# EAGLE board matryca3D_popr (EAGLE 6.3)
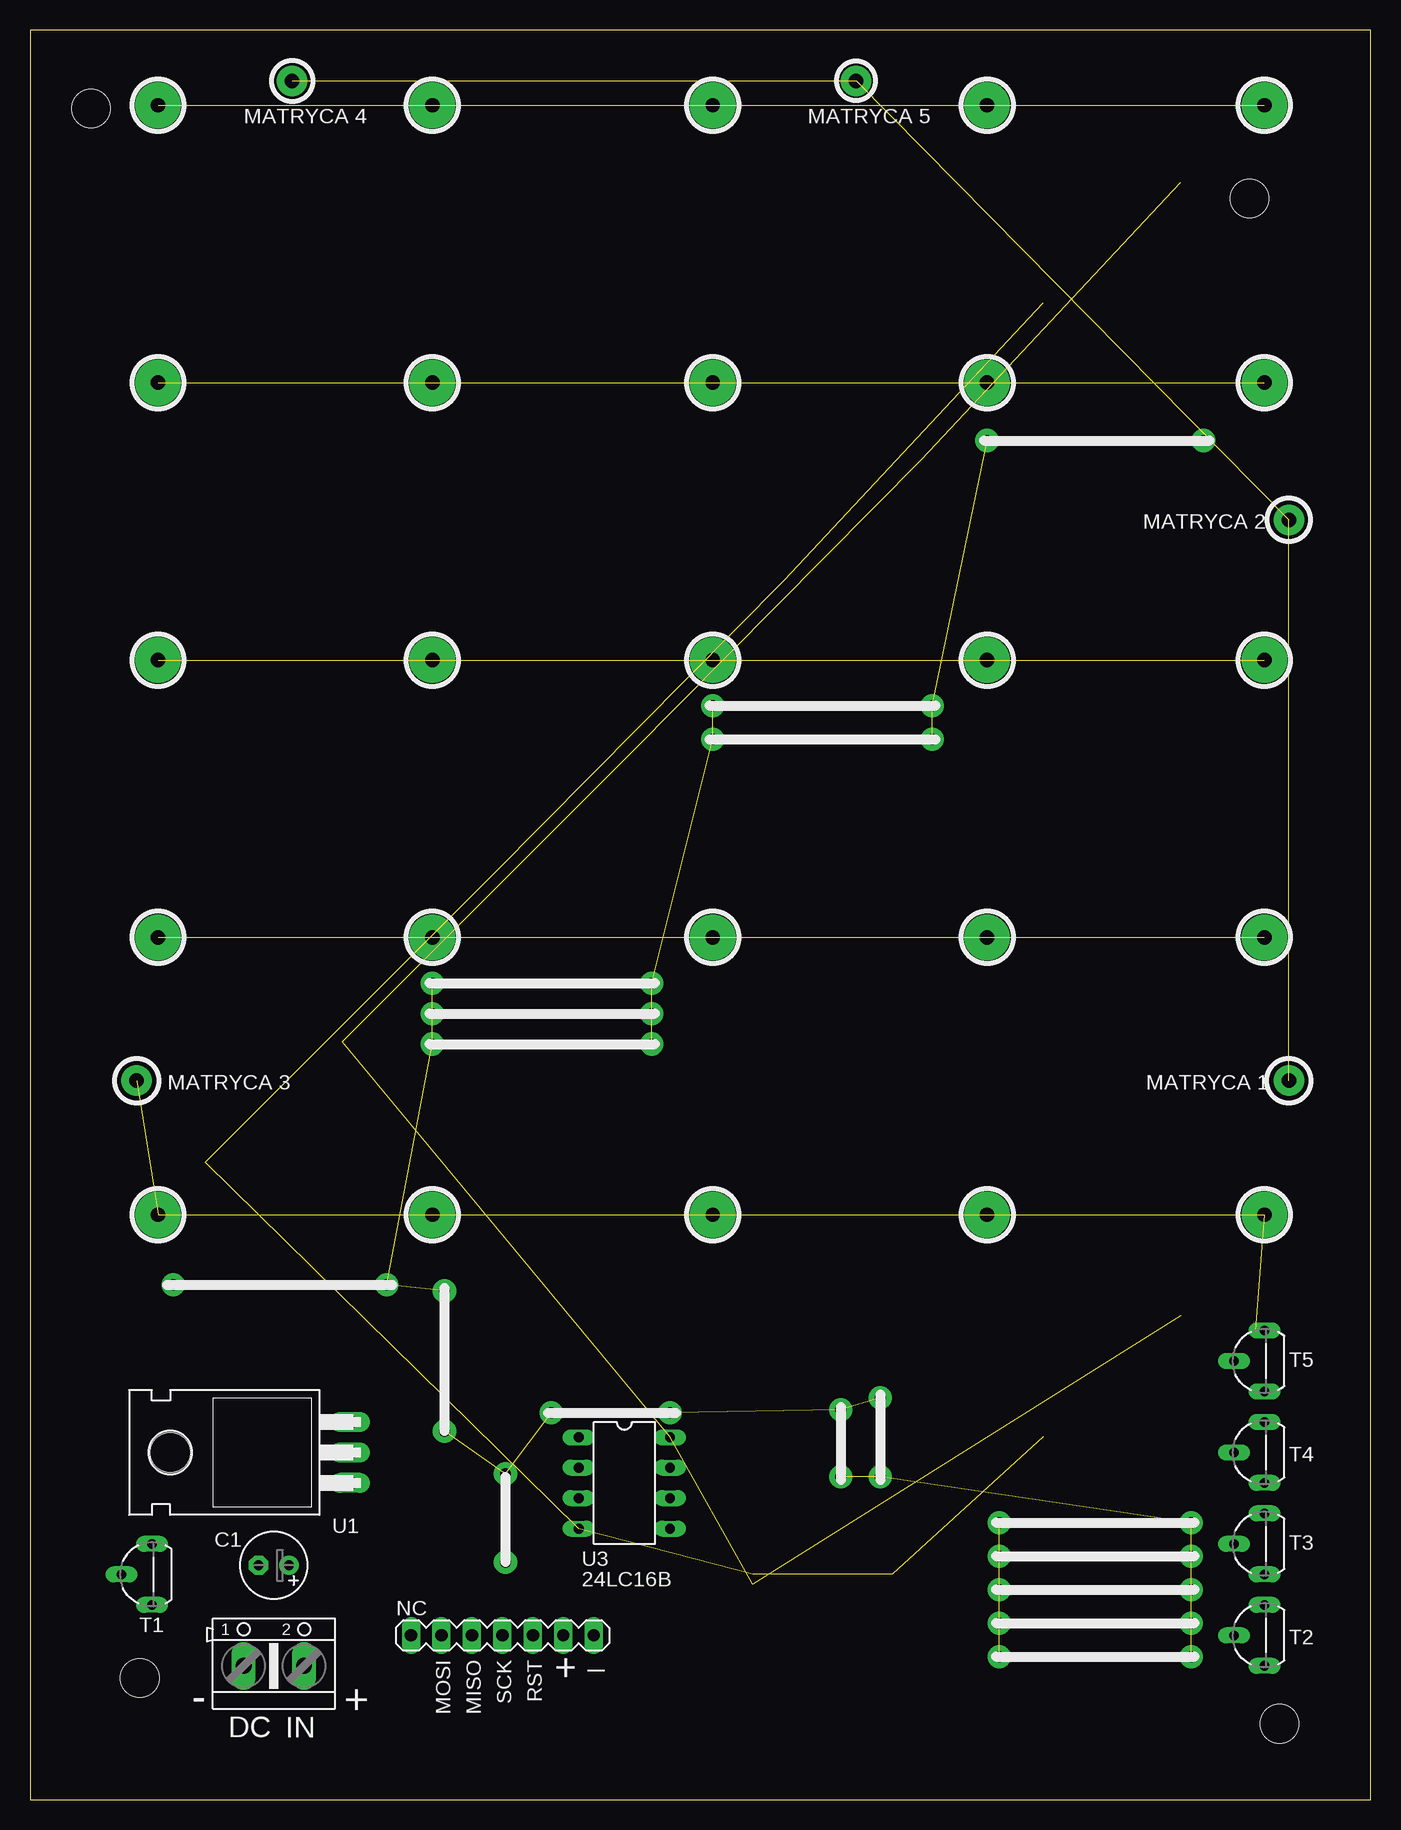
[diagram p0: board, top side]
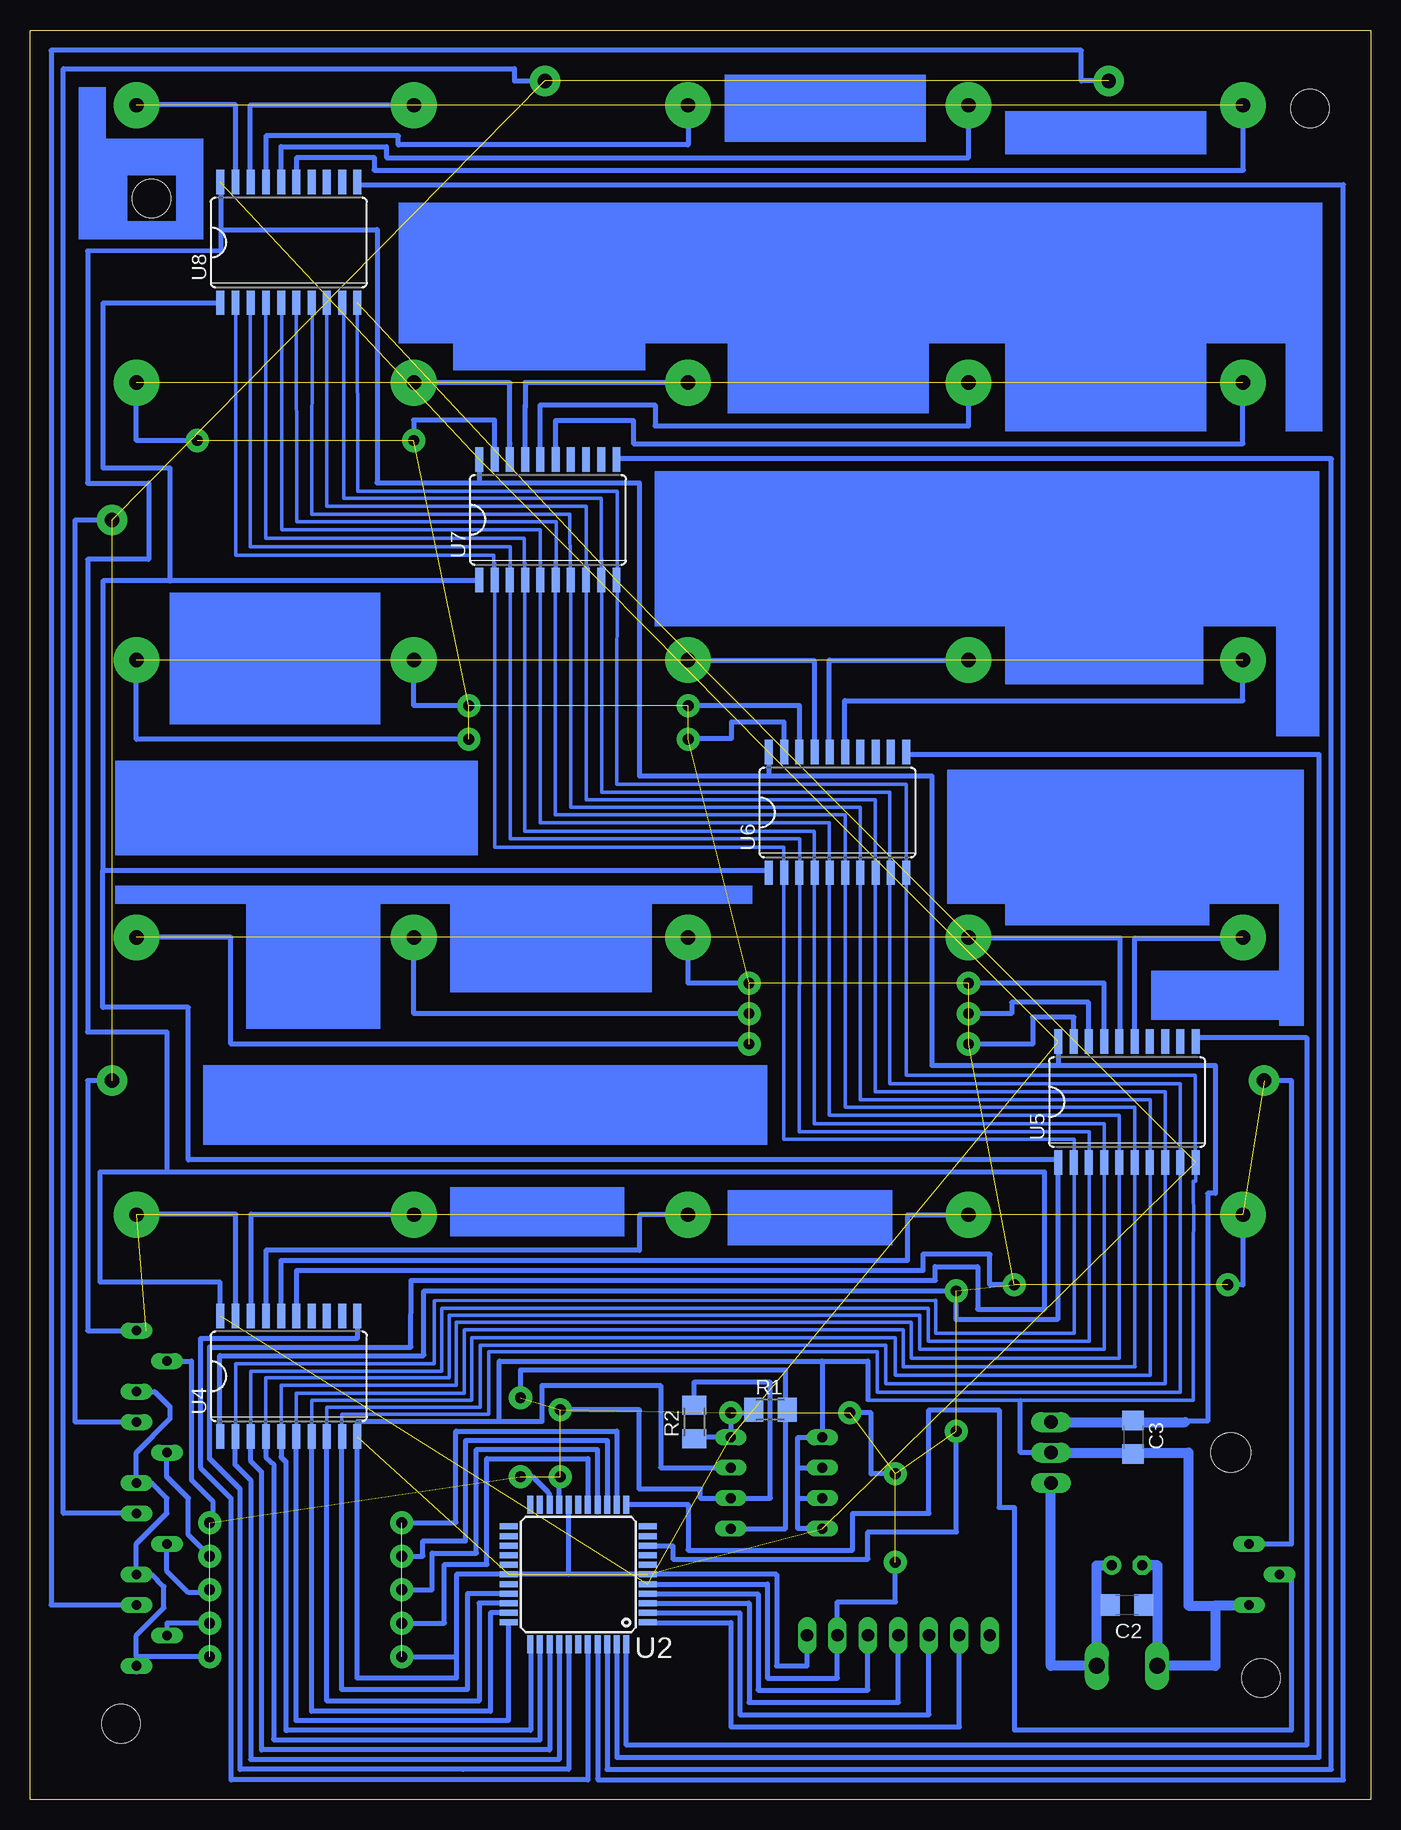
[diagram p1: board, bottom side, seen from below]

Size 111.74 x 147.5 mm. Coordinates in mm from the lower left corner, seen from the top.
Outline: 0,0 111.74,0 111.74,147.5 0,147.5 0,0
Copper layers (1*16): Top 0.035mm / dielectric 1.5mm / Bottom 0.035mm
Design rules "default": minimum track width 10mil, minimum drill 24mil, track to track 8mil, track to pad 8mil, pad to pad 8mil, via to via 8mil, smd to smd 8mil, copper to edge 40mil, drill to drill 8mil, minimum pad ring 10mil, minimum via ring 8mil, stop-mask expansion 4mil, vias tented up to drill 0mil, thermal gap 10mil
Holes 3.2 mm at 9.14,10.16 104.14,6.35 101.63,133.45 5.08,140.97

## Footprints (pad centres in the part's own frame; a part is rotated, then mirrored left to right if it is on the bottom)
E2,5-6 = drill 0.813 pad 1.6: + -1.27,0 | drill 0.813 pad 1.6 octagon: - 1.27,0
C1206 = smd 1.6 x 1.8: 1 -1.4,0; 2 1.4,0
AK500/2 = drill 1.321 long: 1 -2.515,0; 2 2.515,0
MA07-1 = drill 1.016 long: 1 -7.62,0; 2 -5.08,0; 3 -2.54,0; 4 0,0; 5 2.54,0; 6 5.08,0; 7 7.62,0
M1206 = smd 1.6 x 2: 1 -1.4,0; 2 1.4,0
TO92L = drill 0.813 long: 1 0,-2.54; 2 2.54,0; 3 0,2.54
TO220H = drill 1.118 long: 1 -2.54,-10.16; 2 0,-10.16; 3 2.54,-10.16 | hole 3.302: 0,4.826
TQFP44 = smd 1.5 x 0.5: 1 -5.8,4; 2 -5.8,3.2; 3 -5.8,2.4; 4 -5.8,1.6; 5 -5.8,0.8; 6 -5.8,0; 7 -5.8,-0.8; 8 -5.8,-1.6; 9 -5.8,-2.4; 10 -5.8,-3.2; 11 -5.8,-4; 23 5.8,-4; 24 5.8,-3.2; 25 5.8,-2.4; 26 5.8,-1.6; 27 5.8,-0.8; 28 5.8,0; 29 5.8,0.8; 30 5.8,1.6; 31 5.8,2.4; 32 5.8,3.2; 33 5.8,4 | smd 0.5 x 1.5: 12 -4,-5.8; 13 -3.2,-5.8; 14 -2.4,-5.8; 15 -1.6,-5.8; 16 -0.8,-5.8; 17 0,-5.8; 18 0.8,-5.8; 19 1.6,-5.8; 20 2.4,-5.8; 21 3.2,-5.8; 22 4,-5.8; 34 4,5.8; 35 3.2,5.8; 36 2.4,5.8; 37 1.6,5.8; 38 0.8,5.8; 39 0,5.8; 40 -0.8,5.8; 41 -1.6,5.8; 42 -2.4,5.8; 43 -3.2,5.8; 44 -4,5.8
DIL8 = drill 0.813 long: 1 -3.81,-3.81; 2 -1.27,-3.81; 3 1.27,-3.81; 4 3.81,-3.81; 5 3.81,3.81; 6 1.27,3.81; 7 -1.27,3.81; 8 -3.81,3.81
SO20W = smd 0.66 x 2.032: 1 -5.715,-5.029; 2 -4.445,-5.029; 3 -3.175,-5.029; 4 -1.905,-5.029; 5 -0.635,-5.029; 6 0.635,-5.029; 7 1.905,-5.029; 8 3.175,-5.029; 9 4.445,-5.029; 10 5.715,-5.029; 11 5.715,5.029; 12 4.445,5.029; 13 3.175,5.029; 14 1.905,5.029; 15 0.635,5.029; 16 -0.635,5.029; 17 -1.905,5.029; 18 -3.175,5.029; 19 -4.445,5.029; 20 -5.715,5.029

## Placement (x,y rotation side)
C1  [E2,5-6]  20.32,19.56 180 top
C2  [C1206]  20.32,16.26 0 bottom
C3  [C1206]  19.81,30.23 270 bottom
DC  [AK500/2]  20.32,11.18 0 top
NC  [MA07-1]  39.37,13.72 0 top
R1  [M1206]  50.04,32.51 0 bottom
R2  [M1206]  56.39,31.5 90 bottom
T1  [TO92L]  10.16,18.8 180 top
T2  [TO92L]  102.87,13.72 180 top
T3  [TO92L]  102.87,21.34 180 top
T4  [TO92L]  102.87,28.96 180 top
T5  [TO92L]  102.87,36.58 180 top
U1  7805T  [TO220H]  16.51,28.96 90 top
U2  MEGA32-A  [TQFP44]  66.04,18.8 180 bottom
U3  24LC16BP  [DIL8]  49.53,26.42 270 top
U4  74HCT574D  [SO20W]  90.17,35.31 0 bottom
U5  74HCT574D  [SO20W]  20.32,58.17 0 bottom
U6  74HCT574D  [SO20W]  44.45,82.3 0 bottom
U7  74HCT574D  [SO20W]  68.58,106.68 0 bottom
U8  74HCT574D  [SO20W]  90.17,129.79 0 bottom

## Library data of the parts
C1-C3 R1 R2 = rcl
DC = con-ptr500; OC_FARNELL: unknown; OC_NEWARK: unknown
NC = con-lstb; OC_FARNELL: unknown; OC_NEWARK: unknown
T1-T5 = transistor
U1 = linear
U2 = atmel; MPN: ATMEGA32-16AU; OC_FARNELL: 9171274; OC_NEWARK: 69K6677
U3 = microchip; MF: MICROCHIP; MPN: 24LC16B/P; OC_FARNELL: 1200026; OC_NEWARK: 69K7671
U4-U8 = 74xx-eu

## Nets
AVCC: U2.27
GND: U2.6 U2.28 U3.4 U4.10 U5.10 U6.10 U7.10 U8.10
GND1: U2.18
GND2: U2.39
VCC: U2.5 U3.8 U4.20 U5.20 U6.20 U7.20 U8.20
VCC1: U2.17
VCC2: U2.38

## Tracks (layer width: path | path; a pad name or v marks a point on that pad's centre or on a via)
GND  (7 unrouted)
N$1
  Bottom 0.305: 87.02,29.54 87,29.54 87,32.74 74.22,32.74 74.22,37.9 40.41,37.9 40.41,34.67 17.14,34.67 17.14,59 41.3,59 41.3,83.36 65.41,83.36 65.41,102.72
N$2
  Bottom 0.406: 60.48,17.98 50.29,17.98 50.29,10.16 44.45,10.16 44.45,14.73
N$3
  Bottom 0.406: 46.97,12.52 46.99,12.52 46.99,14.73
N$4
  Bottom 0.406: 60.38,17.17 51.05,17.17 51.05,9.14 41.91,9.14 41.91,14.73
N$5
  Bottom 0.406: 60.38,16.41 51.82,16.41 51.82,8.13 39.37,8.13 39.37,14.48
N$6
  Bottom 0.406: 60.43,15.6 52.58,15.6 52.58,7.11 36.83,7.11 36.83,14.73
N$7
  Bottom 0.406: 60.25,14.78 53.34,14.78 53.34,6.1 34.29,6.1 34.29,14.73
N$8  (via drill 0.9 pad 1.93)  (28 unrouted)
  other vias: 39.62,19.81 39.62,27.18 43.43,32.26 34.54,30.73 96.77,23.11 96.77,20.32 96.77,17.53 96.77,14.73 96.77,11.94 79.76,113.28 97.79,113.28 56.9,88.39 56.9,91.19 75.18,91.19 75.18,88.39 33.53,68.07 33.53,65.53 33.53,62.99 51.82,68.07 51.82,65.53 51.82,62.99 67.56,26.92 70.87,26.92 67.56,26.92 67.56,32.51 70.87,33.53 53.34,32.26 34.54,42.42 29.72,42.93 11.94,42.93
N$9
  Bottom 0.305: 89.53,29.84 89.53,33.91 75.56,33.91 75.56,39.17 38.96,39.17 38.96,36.09 19.63,36.09
N$10
  Bottom 0.406: 60.4,21.18 58.17,21.18 58.17,20.07 41.91,20.07 41.91,22.35 34.54,22.35 34.54,31.24
N$11
  Bottom 0.406: 61.98,24.64 56.9,24.64 56.9,20.83 43.18,20.83 43.18,23.88 36.83,23.88 36.83,32.51 30.99,32.51 30.99,24.38 29.72,24.38 29.72,5.84 6.6,5.84 6.6,18.8 8.38,18.8
N$12  (via drill 1.2 pad 3.81)  (4 unrouted)
  other vias: 10.67,141.22 33.53,141.22 56.9,141.22 79.76,141.22 102.87,141.22
N$13
  Bottom 0.813: 10.19,16.2 12.95,16.2 12.95,11.18 17.78,11.18
N$14
  Bottom 0.813: 17.78,11.43 17.78,16.26 | 17.78,16.26 17.78,19.56 | 19.05,16.26 17.78,16.26
N$15
  Bottom 0.813: 17.78,19.56 19.3,19.56
N$16
  Bottom 0.813: 22.81,11.15 22.86,11.15 22.86,19.56 21.34,19.56
N$17
  Bottom 0.813: 21.59,16.26 22.61,16.26
N$18
  Bottom 0.406: 44.48,14.91 44.45,14.91 44.45,16.51 39.62,16.51 39.62,20.32
N$19
  Bottom 0.406: 39.12,27.18 41.66,27.18 41.66,32.26 43.94,32.26
N$20
  Bottom 0.813: 22.35,11.18 26.67,11.18 26.67,26.67
N$21
  Bottom 0.406: 25.4,28.96 29.21,28.96 29.21,33.27
  Bottom 0.813: 27.69,28.96 25.4,28.96 15.21,28.96 15.21,16.2 12.93,16.2
N$22
  Bottom 0.813: 27.69,31.5 15.49,31.5
N$23
  Bottom 0.406: 62.05,13.41 62.05,4.57 5.33,4.57 5.33,63.5 14.48,63.5
N$24
  Bottom 0.406: 62.81,13.49 62.84,13.49 62.84,3.56 4.32,3.56 4.32,87.12 38.71,87.12
N$25
  Bottom 0.406: 63.63,13.46 63.65,13.46 63.65,2.54 3.3,2.54 3.3,111.76 62.99,111.76
N$26
  Bottom 0.406: 64.44,13.39 64.44,1.8 64.41,1.8 64.41,1.68 2.29,1.68 2.29,134.62 84.58,134.62
N$27
  Bottom 0.406: 65.23,13.18 65.25,13.18 65.25,1.68 95,1.68 95,25.15 97.54,27.69 97.54,38.46 84.48,38.46 84.48,41.02
N$28
  Bottom 0.406: 66.85,13.06 66.85,2.54 75.67,2.54
N$29
  Bottom 0.406: 67.64,13.16 67.64,3.35 93.34,3.35
N$30
  Bottom 0.406: 68.45,13.21 68.43,13.21 68.43,4.17 92.43,4.17
N$31
  Bottom 0.406: 69.24,13.16 69.24,4.98 91.39,4.98
N$32
  Bottom 0.406: 70.05,13.16 70.03,13.16 70.03,5.79 90.3,5.79
N$33  (via drill 0.9 pad 1.93)  (4 unrouted)
  other vias: 80.77,23.11 80.77,20.32 80.77,17.53 80.77,14.73 80.77,11.94
N$34
  Bottom 0.406: 96.6,11.94 102.87,11.94 | 102.87,11.94 102.87,10.67 | 102.87,11.94 102.87,13.72 100.58,16 100.58,17.78 101.6,18.8 102.87,18.8 | 102.87,18.8 103.38,18.8 | 102.87,18.8 102.87,21.34 100.33,23.88 100.33,25.15 101.6,26.42 102.87,26.42 | 103.38,26.42 102.87,26.42 | 103.63,34.04 101.35,34.04 100.08,32.77 100.08,31.75 102.87,28.96 102.87,26.42
N$35
  Bottom 0.406: 96.27,17.27 98.55,17.27 100.33,19.05 100.33,21.59
N$36
  Bottom 0.406: 96.27,19.81 98.55,22.1 98.55,25.15 100.33,26.92 100.33,29.21
N$37
  Bottom 0.406: 101.09,36.58 98.3,36.58 98.3,26.67 96.52,24.89 96.52,22.86
N$38
  Bottom 0.406: 102.11,31.5 107.95,31.5 107.95,106.68 103.89,106.68
N$39
  Bottom 0.406: 95.94,30.28 95.91,30.25 95.91,37.03 78.94,37.03
N$40
  Bottom 0.406: 94.67,30.61 94.67,27.96 93.34,26.64 93.34,3.38
N$41
  Bottom 0.406: 93.32,30.76 93.37,30.76 93.37,28.27 92.46,27.36 92.46,4.17
N$42
  Bottom 0.406: 92.05,30.48 92.08,30.48 92.08,28.57 91.44,27.96 91.44,5.08
N$43
  Bottom 0.406: 78.99,37.08 78.92,37.08 78.92,42.42 34.54,42.42
N$44
  Bottom 0.406: 71.88,14.73 71.88,6.6 89.56,6.6 89.56,30.58
N$45
  Bottom 0.406: 96.27,14.73 100.33,14.73 100.33,13.46
N$46
  Bottom 0.406: 71.73,15.6 73.38,15.6 73.38,7.39 88.29,7.39 88.29,30.76 88.27,30.76
N$47
  Bottom 0.406: 71.78,16.41 74.32,16.41 74.32,8.23 87,8.23 87,30.71
N$48
  Bottom 0.305: 92.08,30.58 92.08,35.18 76.81,35.18 76.81,40.41 37.59,40.41 37.59,37.54 29.57,37.54
N$49  (via drill 1.2 pad 3.81)  (4 unrouted)
  other vias: 10.67,118.11 33.53,118.11 56.9,118.11 79.76,118.11 102.87,118.11
N$50  (via drill 1.2 pad 3.81)  (4 unrouted)
  other vias: 10.67,95 33.53,95 56.9,95 79.76,95 102.87,95
N$51  (via drill 1.2 pad 3.81)  (4 unrouted)
  other vias: 10.67,71.88 33.53,71.88 56.9,71.88 79.76,71.88 102.87,71.88
N$52  (via drill 1.2 pad 2.54, 1.2 pad 3.81)  (9 unrouted)
  Bottom 0.406: v104.9,59.94 106.93,59.94 106.93,39.12 102.11,39.12
  other vias: 10.67,48.77 33.53,48.77 56.9,48.77 79.76,48.77 102.87,48.77 8.89,59.94 104.9,106.68 21.84,143.26 68.83,143.26
N$53
  Bottom 0.406: 89.53,135.51 89.51,135.51 89.51,136.88 83.06,136.88 83.06,135.81 10.62,135.81 10.64,142.37
N$54
  Bottom 0.406: 90.81,135.64 90.81,137.77 82.04,137.77 82.04,136.85 33.53,136.85 33.53,142.75
N$55
  Bottom 0.406: 56.87,142.65 56.9,142.65 56.9,137.92 81.05,137.92 81.05,138.68 92.08,138.68 92.08,135.33
N$56
  Bottom 0.406: 93.4,135.46 93.37,135.46 93.37,141.25 78.49,141.25 78.49,141.22
N$57
  Bottom 0.406: 94.61,135.48 94.61,141.25 104.14,141.25 104.14,141.22
N$58
  Bottom 0.406: 67.92,112.75 67.94,112.75 67.94,114.96 61.47,114.96 61.47,113.03 10.67,113.03 10.67,119.38
N$59
  Bottom 0.406: 69.22,111.61 69.22,116.26 59.64,116.26 59.64,114.5 33.53,114.5 33.53,119.38
N$60
  Bottom 0.406: 70.48,112.67 70.48,116.2
N$61
  Bottom 0.406: 55.63,118.11 70.48,118.11 70.48,116
N$62
  Bottom 0.406: 71.73,111.35 71.75,113.03 71.75,118.08 81.31,118.08 81.31,118.03
N$63
  Bottom 0.406: 43.79,88.34 43.84,88.34 43.84,91.62 10.67,91.62 10.67,96.01
N$64
  Bottom 0.406: 45.11,87.45 45.14,86.69 45.14,95 32.26,95
N$65
  Bottom 0.406: 46.35,86.94 46.35,94.92 58.17,94.92 58.17,95
N$66
  Bottom 0.406: 19.74,63.04 19.66,63.04 19.66,71.83 9.14,71.83 9.14,71.88
N$67
  Bottom 0.406: 20.98,62.97 20.9,64.24 20.9,71.83 34.8,71.83 34.8,71.88
N$68
  Bottom 0.406: 82.8,109.75 60.96,109.75 60.96,85.34 36.58,85.34 36.58,61.21 12.95,61.21 12.95,50.55 13.61,50.55 13.61,31.57 15.24,31.57 15.24,31.5
N$69
  Bottom 0.406: 95.76,134.87 95.86,134.87 95.86,130.86 | 95.86,130.86 82.8,130.86 82.8,109.8 | 95.86,130.86 95.86,129.06 106.93,129.08 106.93,109.73 101.85,109.73 101.85,103.38 106.93,103.38 106.93,64.01 100.33,64.01 100.33,52.32 | 75.72,2.54 94.23,2.54 94.23,25.91 96.77,28.45 96.77,37.74 80.01,37.74 79.98,43.31 36.3,43.31 36.32,44.45 32.77,44.45 32.77,40.89 27.18,40.89 27.18,52.32 100.33,52.32 | 100.33,52.32 105.92,52.32 105.92,43.18 95.94,43.18 95.94,39.7
N$70
  Bottom 0.406: 84.45,124.97 84.51,124.97
N$71
  Bottom 0.406: 74.3,112.06 74.32,112.06 74.32,109.78
N$72
  Bottom 0.406: 50.16,87.68 50.16,85.37
N$73
  Bottom 0.406: 26.04,64.06 26.04,61.52
N$74
  Bottom 0.305: 14.61,54 14.61,51.56 14.78,51.56 14.76,47.73 14.78,46.97 14.78,33.33 41.96,33.33
N$75
  Bottom 0.305: 14.63,53.11 14.63,60.4 38.71,60.4 38.71,84.66 62.84,84.66 62.81,109.07 84.43,109.07 84.45,125.45
  Bottom 0.406: 14.61,53.62 14.63,53.11
N$76
  Bottom 0.305: 85.6,125.3 85.6,108.46 64.14,108.46 64.14,103.45 | 64.14,103.45 64.14,102.29 | 64.14,103.45 64.11,103.45 64.11,84 40.08,84 40.08,59.69 15.9,59.69 15.9,33.98 41.15,33.98 41.15,37.34 73.51,37.34 73.51,32.16 85.78,32.16 85.78,29.44
  Bottom 0.406: 85.78,125.3 85.6,125.3 | 71.81,17.2 75.29,17.2 75.29,9.2 85.78,9.2 85.78,29.44 85.78,30.79
N$77
  Bottom 0.305: 65.41,102.79 65.41,107.8 87,107.8 87,125.32
  Bottom 0.406: 65.35,102.79 65.41,102.79
N$78
  Bottom 0.305: 88.24,125.45 88.27,107.16 66.75,107.16 66.73,102.13
  Bottom 0.406: 88.29,125.45 88.24,125.45
N$79
  Bottom 0.305: 67.89,102.13 67.87,106.53 89.51,106.53 89.53,125.09
  Bottom 0.406: 67.92,102.13 67.89,102.13
N$80
  Bottom 0.305: 90.78,125.17 90.78,105.87 69.22,105.87 69.22,102.01
  Bottom 0.406: 90.83,125.17 90.78,125.17
N$81
  Bottom 0.305: 70.48,102.97 70.54,102.97 70.54,105.16 92.1,105.16 92.1,125.42
N$82
  Bottom 0.305: 93.34,125.53 93.4,125.53 93.4,104.42 71.73,104.42 71.73,102.18
N$83
  Bottom 0.305: 72.9,101.85 73.08,101.85 73.08,103.71 94.61,103.71 94.61,125.25
N$84
  Bottom 0.406: 73.03,111.81 73.03,114.99 79.78,114.99 79.78,112.72
N$85
  Bottom 0.406: 97.03,113.28 102.87,113.28 102.87,119.38
N$86
  Bottom 0.406: 34.57,42.88 34.57,40.03 26.11,40.03 26.11,53.34 98.55,53.34 98.55,66.04 105.66,66.04 105.66,77.47 | 105.66,77.47 50.29,77.47 | 74.42,101.6 100.08,101.6 | 100.08,101.6 105.66,101.6 105.66,77.47 | 96.01,124.71 105.66,124.71 105.66,111 100.08,111 100.08,101.6
N$87
  Bottom 0.305: 66.67,102.51 66.67,82.73 42.55,82.73 42.55,58.37 18.39,58.37 18.39,35.38 39.62,35.38 39.62,38.53 74.93,38.53 74.93,33.33 88.27,33.33 88.27,29.92
N$88
  Bottom 0.305: 67.97,103.25 67.97,82.09 43.81,82.09 43.81,57.73 19.66,57.73 19.66,36.09
N$89
  Bottom 0.406: 10.67,50.04 10.67,42.93 12.7,42.93
N$90
  Bottom 0.305: 69.19,103.1 69.22,103.1 69.22,81.43 45.14,81.43 45.14,57.05 20.98,57.05 20.98,36.83 38.3,36.83 38.3,39.8 76.2,39.8 76.2,34.54 90.81,34.54 90.81,29.77 90.93,29.77 90.93,29.72
  Bottom 0.406: 90.81,30.3 90.81,29.77 90.81,28.57 90.42,28.19 90.42,5.79
N$91
  Bottom 0.305: 70.48,103.05 70.51,103.05 70.51,80.75 46.38,80.75 46.38,56.36 22.23,56.36 22.23,37.54 29.62,37.54
N$92
  Bottom 0.305: 71.75,102.79 71.73,102.79 71.7,80.09 47.6,80.09 47.62,55.7 23.47,55.7 23.47,38.23 36.91,38.23 36.88,41 77.42,41 77.44,35.74 93.34,35.74 93.34,29.9
N$93
  Bottom 0.305: 73.05,103.07 73.03,103.07 73.03,79.4 48.92,79.4 48.92,55.04 24.74,55.04 24.74,38.89 36.27,38.89 36.27,41.63 78.05,41.6 78.05,36.35 94.61,36.35 94.61,30
N$94
  Bottom 0.406: 48.9,86.74 48.9,89.81 53.29,89.81 53.29,88.44 57.53,88.44 57.53,88.47
N$95
  Bottom 0.406: 57.56,91.21 47.62,91.21 47.62,87.81
N$96
  Bottom 0.406: 74.42,91.19 79.76,91.19 79.76,96.27
N$97
  Bottom 0.406: 74.68,88.39 102.87,88.39 102.87,96.27
N$98
  Bottom 0.406: 24.77,62.92 24.77,65.25
N$99
  Bottom 0.406: 24.74,65.23 28.19,65.23 28.19,62.99 34.14,62.99
N$100
  Bottom 0.406: 23.47,63.04 23.52,63.04 23.52,66.47 29.95,66.47 29.95,65.53 34.11,65.53 34.11,65.56
N$101
  Bottom 0.406: 22.2,62.92 22.23,62.92 22.23,68.07 34.16,68.07 34.16,68.05
N$102
  Bottom 0.406: 51.31,68.07 56.9,68.07 56.9,72.9
N$103
  Bottom 0.406: 51.31,65.53 79.76,65.53 79.76,73.15
N$104
  Bottom 0.406: 51.05,62.99 95,62.99 95,71.88 104.14,71.88
N$105
  Bottom 0.406: 81.53,14.73 77.22,14.73 77.22,19.63 73.66,19.63 73.66,28.45 65.25,28.45 65.25,24.23
N$106
  Bottom 0.406: 81.53,17.53 78.23,17.53 78.23,20.57 74.55,20.57 74.55,29.21 64.47,29.21 64.47,24
N$107
  Bottom 0.406: 81.53,20.32 78.99,20.32 78.99,21.59 75.44,21.59 75.44,29.97 63.63,29.97 63.63,24.16
N$108
  Bottom 0.406: 81.53,23.11 76.25,23.11 76.25,30.73 62.84,30.73 62.84,24.23
N$109
  Bottom 0.406: 67.64,24.21 67.64,27.51
N$110
  Bottom 0.406: 68.4,24.61 68.45,24.61 68.45,25.5 68.56,25.63 69.85,26.92 71.53,26.92
N$111
  Bottom 0.406: 68.07,32.51 60.96,32.51 60.96,25.91 55.88,25.91 55.88,25.15 50.04,25.15 50.04,34.8 56.39,34.8 56.39,32.51
N$112
  Bottom 0.406: 52.58,27.69 59.18,27.69 59.18,34.54 69.09,34.54 69.09,31.52 72.62,31.52 | 46.99,12.45 46.99,11.18 49.53,11.18 49.53,18.8 66.85,18.8 | 66.85,18.8 66.85,25.02 | 66.85,18.8 76.2,18.8 76.2,11.94 | 76.2,11.94 76.2,10.16 84.48,10.16 84.45,31.52 72.62,31.52 | 81.53,11.94 76.2,11.94 | 72.62,31.52 72.62,36.58 45.72,36.58 | 44.96,22.61 47.75,22.61 47.75,25.15 | 47.75,25.15 47.75,27.69 | 47.75,27.69 47.75,30.23 45.72,30.23 | 45.72,30.23 45.21,30.23 | 47.75,27.69 44.96,27.69 | 47.75,25.15 44.96,25.15 | 45.72,36.58 45.72,30.23 | 45.72,36.58 41.91,36.58 41.91,33.38
N$113
  Bottom 0.406: 54.1,32.26 51.56,32.26 51.56,32.77
N$114
  Bottom 0.406: 53.34,33.02 53.34,29.97
N$115
  Bottom 0.406: 52.58,30.23 56.64,30.23
N$116
  Bottom 0.406: 54.36,22.61 48.77,22.61 48.77,35.81 70.87,35.81 70.87,33.02
N$117
  Bottom 0.406: 29.21,42.93 31.75,42.93 31.75,45.47 37.34,45.47 37.34,44.12 89.53,44.12 89.53,39.57
N$118
  Bottom 0.406: 90.81,39.55 90.81,44.96 38.61,44.96 38.61,48.77 32.26,48.77
N$119
  Bottom 0.406: 55.63,48.77 60.96,48.77 60.96,45.8 92.08,45.8 92.08,39.67
N$120
  Bottom 0.406: 94.61,40.01 94.59,40.01 94.59,48.79 104.22,48.79
N$121
  Bottom 0.406: 93.34,40.06 93.32,40.06 93.32,48.82 78.49,48.82 78.49,48.77
N$122
  Bottom 0.406: 101.85,23.88 108.97,23.88 108.97,144.27 71.37,144.27 71.37,143.26 68.07,143.26
N$123
  Bottom 0.406: 20.83,143.26 24.13,143.26 24.13,145.8 109.98,145.8 109.98,16.26 102.11,16.26
N$124
  Bottom 0.406: 11.18,21.34 6.6,21.34 6.6,59.94 9.65,59.94
VCC  (6 unrouted)
(copper drawn outside any net)
  shapes: Bottom area x28

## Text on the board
tNames: MATRYCA 4 | MATRYCA 5 | MATRYCA 2 | MATRYCA 3 | MATRYCA 1 | 24LC16B | MOSI | MISO | SCK | RST | _ | + | - | + | IN
bStop: KENIC | CUBE LED 5x5x5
